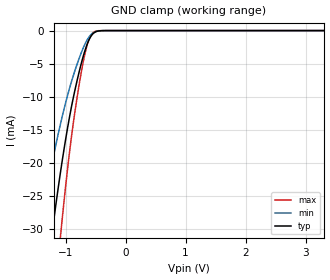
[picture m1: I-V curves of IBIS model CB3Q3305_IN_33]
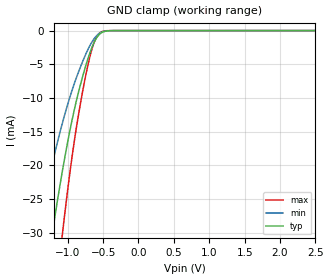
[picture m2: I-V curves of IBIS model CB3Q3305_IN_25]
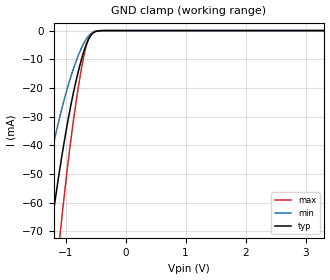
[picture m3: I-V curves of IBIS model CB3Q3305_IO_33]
| TEXAS INSTRUMENTS INCORPORATED
| Standard Linear and Logic Group
| IBIS Model of SN74CB3Q3305
| 2-BIT SWITCH 2.5V/3.3V Low-Voltage FET Bus Switch
| This file contains package information for the following:
|  TSSOP 8-pin (PW) package as [Component] CB3Q3305_PW
| This device can be powered at the following Vccs:
|  3.3 volt Vcc
|  2.5 volt Vcc
| This file provides unique models under the [Model Selector] for each Vcc.
| For operation at a specific Vcc, select the appropriate model after each
| [Model Selector] keyword.
[IBIS Ver]   3.2
[Comment char]  |_char
[File Name]   sn74cb3q3305.ibs
[File Rev]   1.1 | h_die
[Date]   July 14, 2003
[Source]   Data created from TI-SPICE simulations at TI-SLL.
[Notes]   The following is an IBIS list for the CB3Q3305.
   Please contact sllibis@ti.com with questions and
   comments concerning SLL IBIS models.
   - Power-clamp data has been deleted since there is no
   power-clamp diode in the device.
[Disclaimer] Property of Texas Instruments Incorporated.  Unauthorized
   reproduction and/or distribution is strictly prohibited.
   This product is protected under copyright law.
   Created  2003, (C) Copyright  2003, Texas Instruments
   Incorporated, All Rights Reserved
   UNLESS THERE IS A SIGNED, WRITTEN AGREEMENT TO THE
   CONTRARY, TEXAS INSTRUMENTS (TI) IS PROVIDING THE IBIS
   MODELS  AND WITHOUT ANY WARRANTY, EXPRESSED OR
   IMPLIED.  TI assumes no liability for:
   1) the accuracy of the IBIS models provided to your
   company;
   2) the proper functioning of these IBIS Models in your
   design or for any resulting applications; or
   3) infringement of patents, copyrights or intellectual
   property rights resulting from your use of these IBIS
   models.
   TI provides IBIS Models as a service to our customers.
   You and your company shall not distribute, sell or give
   these models to anyone else without prior written
   permission from TI.
   TI reserves the right to make changes to our products or
   to discontinue any semiconductor product or service
   without notice, and advises our customers to obtain the
   latest version of relevant information to verify, before
   placing orders, that the information being relied on is
   current.
   Please be aware that your receipt and use of the IBIS
   information provided shall serve as acceptance of these
   terms and conditions.  If you do not accept these terms,
   you should return or destroy the IBIS models and any
   other accompanying information immediately.
| Component CB3Q3305_PW 8-pin TSSOP
[Component]   CB3Q3305_PW
[Manufacturer]   Texas Instruments, Inc.
[Package]
|   typ   min   max
R_pkg   4.000e-02   3.400e-02   4.600e-02
L_pkg   2.625e-09   2.419e-09   2.861e-09
C_pkg   3.040e-13   2.860e-13   3.210e-13
[Pin]   signal_name   model_name   R_pin   L_pin   C_pin
1   1OE   CB3Q3305_IN   4.600e-02   2.861e-09   3.210e-13
2   1A   CB3Q3305_IO   3.700e-02   2.437e-09   2.860e-13
3   1B   CB3Q3305_IO   3.400e-02   2.419e-09   2.860e-13
4   GND   GND   4.300e-02   2.784e-09   3.210e-13
5   2A   CB3Q3305_IO   4.300e-02   2.784e-09   3.210e-13
6   2B   CB3Q3305_IO   3.500e-02   2.420e-09   2.860e-13
7   2OE   CB3Q3305_IN   3.700e-02   2.437e-09   2.860e-13
8   VCC   POWER   4.600e-02   2.860e-09   3.210e-13
[Series Switch Groups]
| Function Group States
On  1 /   | 1a->1b 1oe high
On  2 /   | 2a->2b 2oe high
On  1 2 /   | enable both
Off 1 2  /   | 1oe low, 2oe low, disable both
[Series Pin Mapping]   pin_2   model_name   function_table_group
2   3   CB3Q3305_IO_33_S   1
| 2   3   CB3Q3305_IO_25_S   1
5   6   CB3Q3305_IO_33_S   2
| 5   6   CB3Q3305_IO_25_S   2
| Model CB3Q3305_IN
[Model Selector]   CB3Q3305_IN
CB3Q3305_IN_33   3.3 volt Vcc
CB3Q3305_IN_25   2.5 volt Vcc
| Model CB3Q3305_IO
[Model Selector]   CB3Q3305_IO
CB3Q3305_IO_33   3.3 volt Vcc
CB3Q3305_IO_25   2.5 volt Vcc
| Model CB3Q3305_IO_S
[Model Selector]   CB3Q3305_IO_S
CB3Q3305_IO_33_S   3.3 volt Vcc_S
CB3Q3305_IO_25_S   2.5 volt Vcc_S
[Model]   CB3Q3305_IO_33_S
Model_type  Series_switch
| variable   typ   min   max
C_comp   0   0   0
[Temperature Range]   40   100   -40
| Ambient temperature   25   85   -40
[Voltage range]   3.3   3   3.6
[On]
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[Off]
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[Model]   CB3Q3305_IO_25_S
Model_type  Series_switch
| variable   typ   min   max
C_comp   0   0   0
[Temperature Range]   40   100   -40
| Ambient temperature   25   85   -40
[Voltage range]   2.5   2.3   2.7
[On]
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[Off]
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| Models and submodels in the file (6): CB3Q3305_IN_33 (Input), CB3Q3305_IN_25 (Input), CB3Q3305_IO_33_S (Series_switch), CB3Q3305_IO_33 (Terminator), CB3Q3305_IO_25_S (Series_switch), CB3Q3305_IO_25 (Terminator)
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[Model]   CB3Q3305_IN_33
Model_type  Input
Vinl=0.8
Vinh=2.0
| variable   typ   min   max
C_comp   2.92pF   2.24pF   4.26pF
[Temperature Range]   40   100   -40
| Ambient temperature   25   85   -40
[Voltage range]   3.3   3   3.6
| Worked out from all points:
|   GND clamp passes 1 mA (typ) near -0.59 V on its own axis
[GND Clamp]
| CB3Q3305_IN_33
|   Voltage   I(typ)   I(min)   I(max)
-5.5V     -472.5mA   -358.4mA   -595mA
-1.435V   -46.41mA   -30.52mA   -67.59mA
-1.225V   -30.63mA   -20.08mA   -44.85mA
-1.085V   -21.45mA   -14.13mA   -31.14mA
-1.065V   -20.24mA   -13.35mA   -29.31mA
-980mV    -15.43mA   -10.26mA   -21.99mA
-905mV    -11.68mA   -7.824mA   -16.3mA
-775mV    -6.3mA     -4.241mA   -8.247mA
-655mV    -2.433mA   -1.648mA   -2.666mA
-595mV    -1.146mA   -802.4uA   -1.007mA
-535mV    -406.3uA   -315.1uA   -250.7uA
3.3V      128.8pA    501.8pA    26.94pA
[Model]   CB3Q3305_IN_25
Model_type  Input
Vinl=0.7
Vinh=1.7
| variable   typ   min   max
C_comp   2.39pF   1.91pF   2.60pF
[Temperature Range]   40   100   -40
| Ambient temperature   25   85   -40
[Voltage range]   2.5   2.3   2.7
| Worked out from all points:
|   GND clamp passes 1 mA (typ) near -0.59 V on its own axis
[GND Clamp]
| CB3Q3305_IN_25
|   Voltage   I(typ)   I(min)   I(max)
-5.5V     -472.5mA   -358.4mA   -595mA
-1.425V   -45.61mA   -29.98mA   -66.47mA
-1.205V   -29.25mA   -19.18mA   -42.81mA
-1.07V    -20.54mA   -13.54mA   -29.76mA
-930mV    -12.88mA   -8.603mA   -18.1mA
-785mV    -6.676mA   -4.493mA   -8.803mA
-725mV    -4.527mA   -3.05mA    -5.644mA
-655mV    -2.433mA   -1.648mA   -2.666mA
-605mV    -1.323mA   -917.7uA   -1.217mA
-550mV    -542.1uA   -406.5uA   -369.1uA
-350mV    -3.742uA   -5.539uA   -427.8nA
2.5V      96.07pA    415.1pA    20.34pA
[Model]   CB3Q3305_IO_33
Model_type  Terminator
| variable   typ   min   max
C_comp   4.06pF   3.45pF   5.22pF
| C_tri-state   4.06pF   3.45pF   5.22pF
[Temperature Range]   40   100   -40
| Ambient temperature   25   85   -40
[Voltage range]   3.3   3   3.6
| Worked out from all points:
|   GND clamp passes 1 mA (typ) near -0.55 V on its own axis
[GND Clamp]
| CB3Q3305_IO_33
|   Voltage   I(typ)   I(min)   I(max)
-5.5V     -1.002A    -757.8mA   -1.259A
-1.485V   -109.2mA   -69.97mA   -160mA
-1.245V   -69.78mA   -43.93mA   -104mA
-1.095V   -48.22mA   -30.06mA   -72.04mA
-1.075V   -45.57mA   -28.37mA   -68.03mA
-915mV    -26.42mA   -16.3mA    -38.75mA
-830mV    -18.01mA   -11.01mA   -25.72mA
-755mV    -11.61mA   -7.024mA   -15.66mA
-650mV    -4.604mA   -2.799mA   -5.005mA
-555mV    -1.109mA   -775.3uA   -764.8uA
-330mV    -3.637uA   -5.843uA   -333.9nA
3.3V      197.8pA    862.6pA    19.5pA
